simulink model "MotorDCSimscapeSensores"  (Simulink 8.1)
settings: Solver=ode45  StartTime=0.0  StopTime=tmax  MaxStep=1e-4  RelTol=1e-3
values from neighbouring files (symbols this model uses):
  Jm = 1.4e-6    (= 1.4e-06)    [MotorDCParam.m]
  K1 = 1/(2*pi)    (= 0.159154943092)    [MotorDCParam.m]
  K2 = 1/25    (= 0.04)    [MotorDCParam.m]
  K3 = 10    [MotorDCParam.m]
  U = 5    [MotorDCParam.m]
libraries: fl_lib x5, nesl_utility x5, elec_lib x1

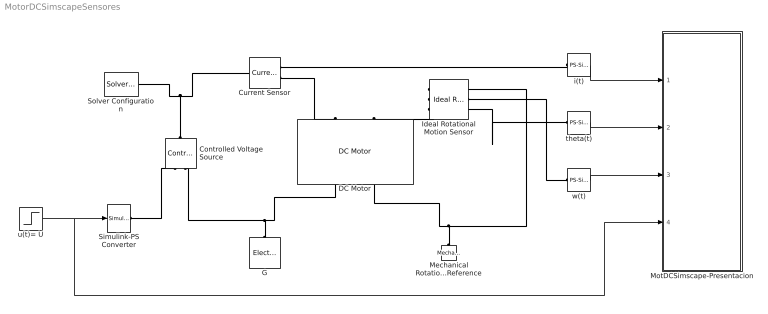
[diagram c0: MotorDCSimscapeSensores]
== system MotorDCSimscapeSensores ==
  Controlled Voltage Source : fl_lib/Electrical/Electrical Sources/Controlled Voltage Source  i_Log=off  v_Log=off  LocalVarNames=|i|v  LocalVarDescs=|i|v  LocalVarLogging=[0 0]
  Current Sensor : fl_lib/Electrical/Electrical Sensors/Current Sensor  i1_Log=off  v1_Log=off  LocalVarNames=|i1|v1  LocalVarDescs=|i1|v1  LocalVarLogging=[0 0]
  DC Motor : elec_lib/Actuators & Drivers/Rotational Actuators/DC Motor  parameterization=1  Ra=Rm Ohm  La=Lm H  emf_or_torque=1  Kv=kb V/(rad/s)  Ki=6.876e-4 N*m/A  T_stall=2.4e-4 N*m  w_max=1.91e+4 rpm  w_rated=1.5e+4 rpm  P_rated=0.08 W  V_rated=1.5 V  J=Jm kg*m^2  lam_param=1  lam=Bm N*m/(rad/s)  i_noload=0 A  V_i_noload=1.5 V  speed0=0 rad/s  current_Log=off  voltage_Log=off  power_Log=off  i2r_Log=off  torque_Log=off  speed_Log=off  LocalVarNames=|current|voltage|power|i2r|torque|speed  LocalVarDescs=|Current (A)|Voltage (V)|Power (W)|Electrical losses (W)|Torque (Nm)|Angular speed (rad/s)  LocalVarLogging=[0 0 0 0 0 0]  alpha=0.00393 1/K  Tmeas=25 C  thermal_mass=100 J/K  initial_temperature=25 C
  G : fl_lib/Electrical/Electrical Elements/Electrical Reference  i_Log=off  LocalVarNames=|i  LocalVarDescs=|i  LocalVarLogging=0
  Ideal Rotational Motion Sensor : fl_lib/Mechanical/Mechanical Sensors/Ideal Rotational Motion Sensor  offset=0 rad  w_Log=off  t_Log=off  phi_Log=off  LocalVarNames=|w|t|phi  LocalVarDescs=|w|t|phi  LocalVarLogging=[0 0 0]
  Mechanical Rotational Reference : fl_lib/Mechanical/Rotational Elements/Mechanical Rotational Reference  t_Log=off  LocalVarNames=|t  LocalVarDescs=|t  LocalVarLogging=0
  MotDCSimscape-Presentacion : Subsystem
  Simulink-PS Converter : nesl_utility/Simulink-PS Converter  PhysicalDomain=network_engine_domain  SubClassName=ps_input  LeftPortType=input  RightPortType=output  PseudoPeriodic=off  Frequencies=[]  NoiseDistribution=none  NoiseParameters=[]  Unit=V  AffineConversion=off  InputFiltering=off  SimscapeFilterOrder=1  InputFilterTimeConstant=0.001  UdotUserProvided=2
  Solver Configuration : nesl_utility/Solver Configuration  PhysicalDomain=network_engine_domain  SubClassName=solver  LeftPortType=input  RightPortType=generic  Accelerate=off  Tones=[]  Harmonics=[]  SimulateNoise=off  Profile=off  UseLocalSampling=off  EnableSwitchedLinearOptims=on  FrequencyDomain=off  UseCCode=off  UseNewInitialization=off  DoDC=off  ResidualTolerance=1e-9  UseLocalSolver=off  LocalSolverChoice=NE_BACKWARD_EULER_ADVANCER  LocalSolverSampleTime=0.001  DoFixedCost=off  MaxNonlinIter=3  MaxModeIter=2  LinearAlgebra=Sparse  DelaysMemoryBudget=1024
  i(t) : nesl_utility/PS-Simulink Converter  PhysicalDomain=network_engine_domain  SubClassName=ps_output  LeftPortType=input  RightPortType=output  PseudoPeriodic=off  Frequencies=[]  Unit=A  AffineConversion=off
  theta(t) : nesl_utility/PS-Simulink Converter  PhysicalDomain=network_engine_domain  SubClassName=ps_output  LeftPortType=input  RightPortType=output  PseudoPeriodic=off  Frequencies=[]  Unit=rad  AffineConversion=off
  u(t)= U : Step  Time=0  After=U  SampleTime=0
  w(t) : nesl_utility/PS-Simulink Converter  PhysicalDomain=network_engine_domain  SubClassName=ps_output  LeftPortType=input  RightPortType=output  PseudoPeriodic=off  Frequencies=[]  Unit=rad/s  AffineConversion=off
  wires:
  i(t)/1 -> MotDCSimscape-Presentacion/1(i(t))
  theta(t)/1 -> MotDCSimscape-Presentacion/2(theta(t))
  w(t)/1 -> MotDCSimscape-Presentacion/3("w(t) ")
  u(t)= U/1 -> MotDCSimscape-Presentacion/4(u(t)), Simulink-PS Converter/1
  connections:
  Mechanical Rotational Reference/LConn1 -- Ideal Rotational Motion Sensor/RConn1 -- DC Motor/RConn2
  Controlled Voltage Source/LConn1 -- Current Sensor/LConn1 -- Solver Configuration/RConn1
  Ideal Rotational Motion Sensor/RConn3 -- theta(t)/LConn1
  w(t)/LConn1 -- Ideal Rotational Motion Sensor/RConn2
  Simulink-PS Converter/RConn1 -- Controlled Voltage Source/RConn1
  G/LConn1 -- Controlled Voltage Source/RConn2 -- DC Motor/RConn1
  i(t)/LConn1 -- Current Sensor/RConn1
  Current Sensor/RConn2 -- DC Motor/LConn1
  Ideal Rotational Motion Sensor/LConn1 -- DC Motor/LConn2

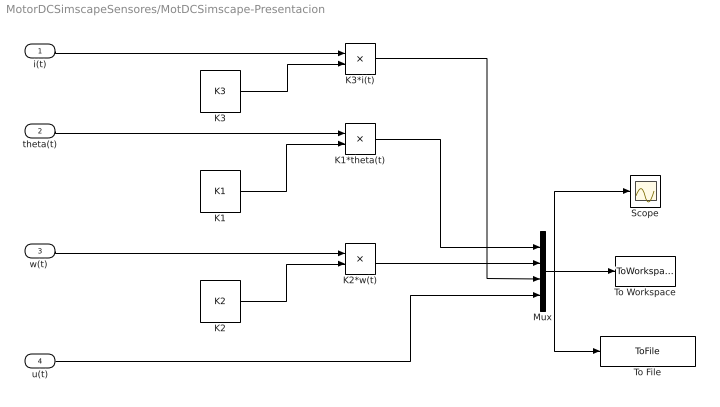
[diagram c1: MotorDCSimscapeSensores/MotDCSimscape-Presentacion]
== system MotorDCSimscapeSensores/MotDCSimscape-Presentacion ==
  i(t) : Inport
  theta(t) : Inport  Port=2
  "w(t) " : Inport  Port=3
  u(t) : Inport  Port=4
  K1 : Constant  Value=K1
  K1*theta(t) : Product
  K2 : Constant  Value=K2
  K2*w(t) : Product
  K3 : Constant  Value=K3
  K3*i(t) : Product
  Mux : Mux
  Scope : Scope
  To File : ToFile  Filename=Mot.mat  SaveFormat=Timeseries
  To Workspace : ToWorkspace  VariableName=Mot  SampleTime=-1
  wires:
  K2/1 -> K2*w(t)/2
  K2*w(t)/1 -> Mux/2
  Mux/1 -> To File/1, To Workspace/1, Scope/1
  theta(t)/1 -> K1*theta(t)/1
  K1*theta(t)/1 -> Mux/1
  K1/1 -> K1*theta(t)/2
  i(t)/1 -> K3*i(t)/1
  "w(t) "/1 -> K2*w(t)/1
  u(t)/1 -> Mux/4
  K3*i(t)/1 -> Mux/3
  K3/1 -> K3*i(t)/2
